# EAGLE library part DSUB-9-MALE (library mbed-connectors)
DSUB Connector male 9-pol
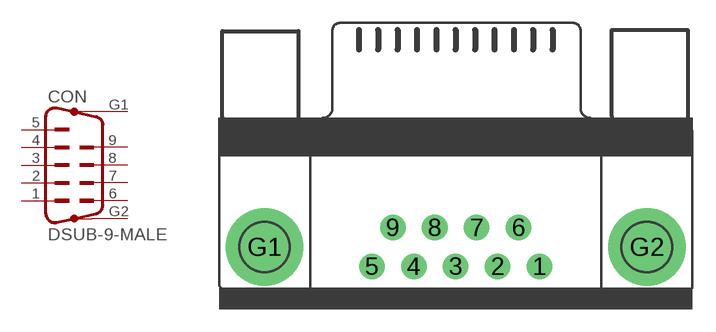
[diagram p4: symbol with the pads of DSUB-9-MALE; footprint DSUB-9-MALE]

Designator prefix CON

## DSUB-9-MALE  [DSUB-9-MALE]
1  5  pas
2  4  pas
3  3  pas
4  2  pas
5  1  pas
6  9  pas
7  8  pas
8  7  pas
9  6  pas
G1  G1  pas
G2  G2  pas

## Footprint DSUB-9-MALE (pad centres in mm)
DSUB Connector male 9-pol
drill 1.016 pad 1.676: 1 5.486,-1.524; 2 2.743,-1.524; 3 0,-1.524; 4 -2.743,-1.524; 5 -5.486,-1.524; 6 4.115,1.016; 7 1.372,1.016; 8 -1.372,1.016; 9 -4.115,1.016
drill 3.302 pad 5.08: G1 -12.522,-0.254; G2 12.522,-0.254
